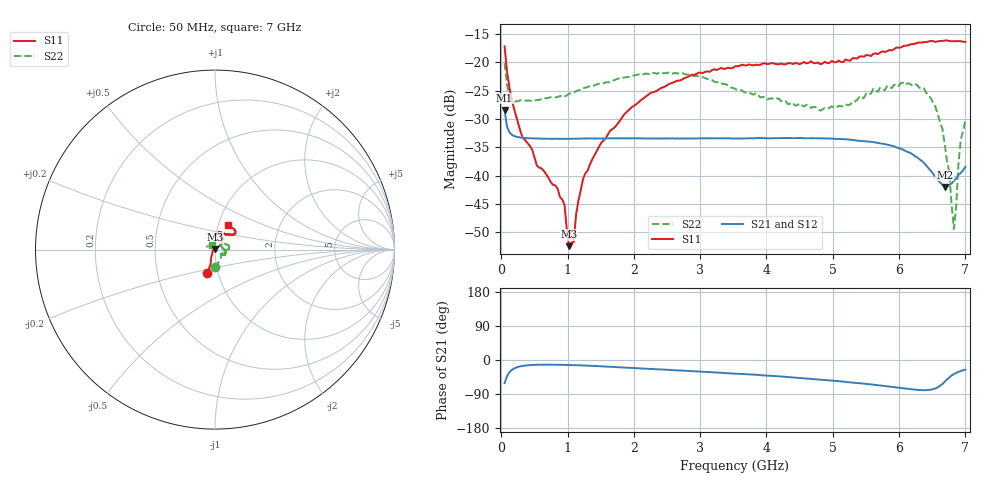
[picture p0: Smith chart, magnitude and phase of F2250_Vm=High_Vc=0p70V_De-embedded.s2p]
! Integrated Device Technology
! Corporate Headquarters
! 6024 Silver Creek Valley Road
! San Jose, CA 95138  USA
! Phone:  1-408-284-8200
! Toll Free:  1-800-223-1366
! Webpage:  http://www.idt.com/
! Timing and RF Division
! 515 Groton Road, Suite 102
! Westford, MA 01886-6024
! Device:  F2250
! Description: Voltage Variable RF Attenuator
! Frequency:  50.0 -  6000.00 MHz
! Package:  3x3 mm Thin QFN Plastic Package: 16 pin
! Ports:  2 RF, 3 DC
!  Pin  1  = GND
!  Pin  2  = NC
!  Pin  3  = RF1  = Port 1
!  Pin  4  = NC
!  Pin  5  = GND
!  Pin  6  = GND
!  Pin  7  = GND
!  Pin  8  = GND
!  Pin  9  = NC
!  Pin 10  = RF2  = Port 2
!  Pin 11  = NC
!  Pin 12  = GND
!  Pin 13  = GND
!  Pin 14  = VCNTRL
!  Pin 15  = VDD
!  Pin 16  = VMODE
! Vcntrl:  0.700 Volts
! Vmode:  +3.300 Volts
! Vdd:  +3.30  Volts
! Current:  1.288 mA
! Data:  The device was measured on a the F2250 evaluation board which has
!  individual transmission lines to the RF pins.  Data was collected
!  using a calibrated network analyzer.  The evaluation board was
!  de-embedded using a TRL calibration technique.
!  The reference plane is the edge of the package pin.
! Misc:  SN 10
!  Action Tracker AT0258
! Date Measured:  2014-11-26
! Date:  2015-10-15  MJV
! Note:
!  Integrated Device Technology supplies this data as a sample of measured
!  data at the package pin for this product.  Your particular data for this
!  product may vary.
!  Data was taken at 25 degrees C.
!  Integrated Device Technology reserves the right to change this data at anytime.
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# GHz S dB R 50
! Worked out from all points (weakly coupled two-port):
!   201 points, 50 MHz to 7 GHz, reference 50 ohm
!   highest |S21| = -28.40 dB at 50 MHz (marker M1); lowest = -42.0 dB at 6.687 GHz (marker M2)
!   lowest |S11| = -52.4 dB at 1.023 GHz (marker M3), VSWR 1.00, Z = 49.8 + j0.166 ohm
!   |S11| at or under -10 dB: start of sweep to end of sweep
!   |S22| runs from -49.4 to -20.1 dB; largest |S21 - S12| = 6.7e-05
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0.05  -17.16 -108.1  -28.40 -61.1  -28.39 -61.1  -20.11 -91.0
0.1195  -24.20 -111.3  -32.26 -32.9  -32.27 -33.0  -25.75 -48.4
0.29325  -32.34 -126.2  -33.27 -16.5  -33.27 -16.6  -26.63 -20.5
0.9535  -45.10 171.8  -33.48 -12.9  -33.49 -12.9  -25.98 -6.1
1.023  -52.43 135.9  -33.48 -13.2  -33.48 -13.2  -25.53 -5.2
1.0925  -51.71 78.1  -33.47 -13.5  -33.47 -13.5  -25.31 -4.6
1.12725  -46.97 54.8  -33.48 -13.7  -33.47 -13.7  -25.08 -5.1
1.2315  -40.61 37.5  -33.44 -14.4  -33.44 -14.3  -24.60 -5.7
1.6485  -31.96 40.1  -33.40 -17.8  -33.40 -17.8  -23.40 -0.7
2.37825  -24.75 46.1  -33.41 -24.7  -33.42 -24.7  -21.85 7.8
3.525  -20.69 71.4  -33.42 -35.9  -33.42 -35.9  -24.64 30.9
4.7065  -20.10 71.8  -33.38 -50.1  -33.38 -50.1  -27.85 38.0
5.2625  -19.69 53.0  -33.63 -59.1  -33.62 -59.1  -27.44 9.5
5.85325  -17.81 40.4  -34.62 -70.1  -34.60 -70.3  -24.22 -14.5
6.3745  -16.42 40.8  -37.73 -79.7  -37.75 -79.7  -24.57 -30.4
6.54825  -16.36 44.5  -40.18 -75.0  -40.19 -75.0  -27.84 -38.4
6.68725  -16.13 47.7  -41.99 -57.6  -41.98 -57.7  -34.34 -32.4
6.75675  -16.21 50.4  -41.62 -46.6  -41.61 -46.6  -39.30 -33.2
6.82625  -16.25 52.4  -40.89 -37.3  -40.85 -37.4  -49.39 99.5
6.861  -16.24 54.3  -40.47 -33.9  -40.45 -34.0  -45.40 116.0
6.9305  -16.25 58.6  -39.50 -29.2  -39.47 -29.4  -33.63 127.4
7  -16.36 62.3  -38.43 -25.7  -38.40 -25.9  -30.15 128.8
